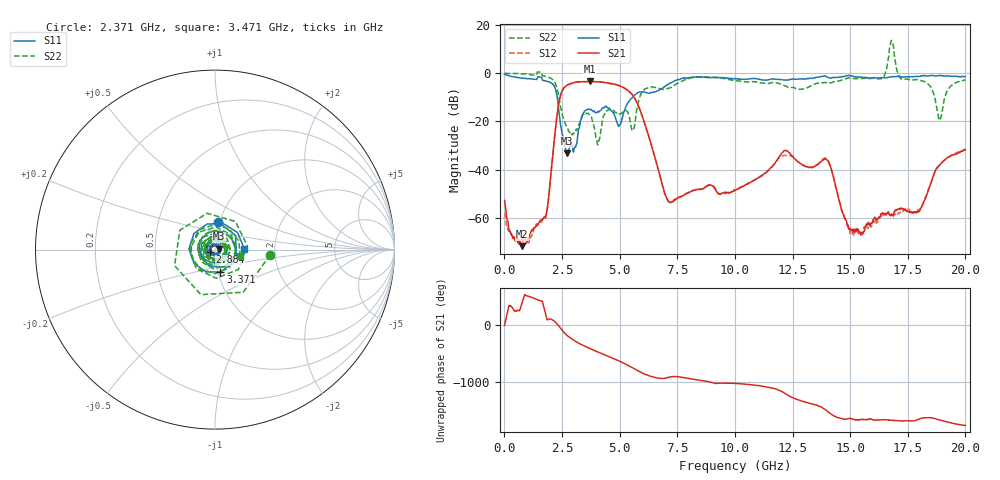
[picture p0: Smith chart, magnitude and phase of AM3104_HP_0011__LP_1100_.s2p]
!Created with skrf (http://scikit-rf.org).
# Hz S RI R 50.0
!freq ReS11 ImS11 ReS21 ImS21 ReS12 ImS12 ReS22 ImS22
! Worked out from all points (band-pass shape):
!   1601 points, 10 MHz to 20 GHz, reference 50 ohm
!   highest |S21| = -3.39 dB at 3.708 GHz (marker M1); lowest = -71.7 dB at 772.1 MHz (marker M2)
!   |S21| within 3 dB of the highest: 2.561 GHz to 5.256 GHz (2.695 GHz wide, 68.9 % of centre)
!   lowest |S11| = -33.3 dB at 2.709 GHz (marker M3), VSWR 1.04, Z = 52.2 + j0.475 ohm
!   |S11| at or under -10 dB: 2.295 GHz to 5.559 GHz (3.264 GHz wide, 83.1 % of centre)
!   |S22| runs from -29.7 to 13.6 dB; largest |S21 - S12| = 0.058
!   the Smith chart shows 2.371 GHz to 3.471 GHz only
!   S11 on the Smith chart (normalised r, x): 2.371 GHz: 0.98, +0.31; 2.884 GHz: 0.94, -0.03; 3.371 GHz: 1.03, -0.26; 3.471 GHz: 1.39, +0.01
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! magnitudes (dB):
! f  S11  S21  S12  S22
! 10 MHz  -0.4  -52.8  -57.9  0.0
! 772.1 MHz  -2.0  -71.7  -68.4  -0.2
! 1.797 GHz  -3.2  -58.9  -59.8  -1.3
! 2.371 GHz  -16.1  -12.0  -12.0  -10.2
! 2.709 GHz  -33.3  -5.0  -5.0  -22.3
! 2.884 GHz  -29.6  -4.2  -4.3  -25.3
! 3.346 GHz  -18.6  -3.5  -3.6  -18.3
! 3.371 GHz  -17.8  -3.5  -3.6  -17.5
! 3.471 GHz  -15.8  -3.5  -3.5  -16.7
! 3.708 GHz  -15.1  -3.4  -3.5  -17.7
! 5.545 GHz  -10.2  -8.9  -8.8  -23.8
! 6.682 GHz  -7.2  -40.2  -40.1  -6.2
! 7.181 GHz  -4.1  -53.6  -53.7  -6.0
! 10.01 GHz  -2.4  -48.7  -48.7  -3.1
! 12.17 GHz  -2.8  -32.1  -34.0  -5.2
! 13.34 GHz  -2.1  -39.1  -39.0  -5.0
! 14.03 GHz  -1.7  -36.2  -36.1  -4.0
! 15.09 GHz  -1.1  -64.7  -66.5  -2.1
! 16.68 GHz  -1.6  -57.8  -58.3  7.3
! 18 GHz  -1.3  -57.3  -56.8  -2.9
! 18.89 GHz  -1.0  -38.0  -38.0  -19.4
! 20 GHz  -1.3  -31.7  -31.5  -2.8
